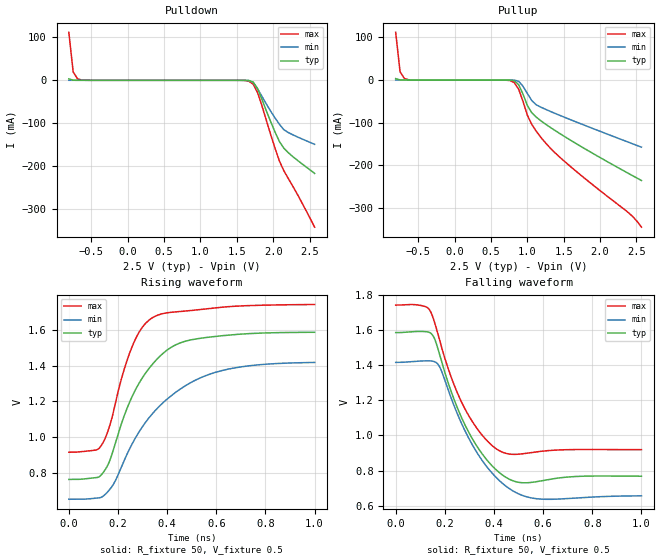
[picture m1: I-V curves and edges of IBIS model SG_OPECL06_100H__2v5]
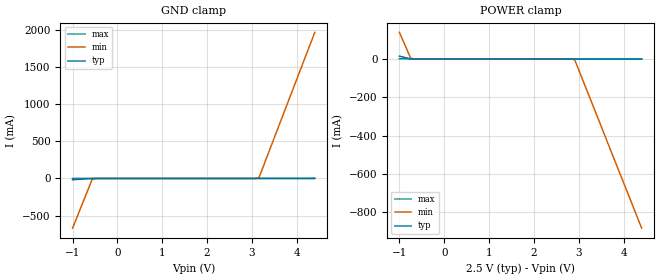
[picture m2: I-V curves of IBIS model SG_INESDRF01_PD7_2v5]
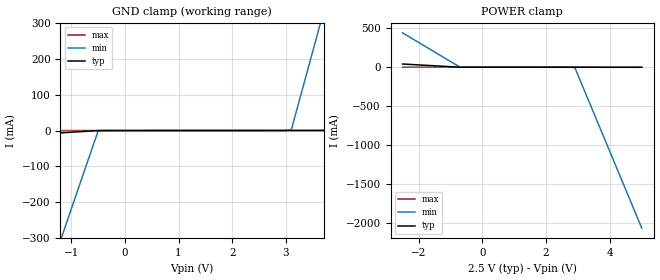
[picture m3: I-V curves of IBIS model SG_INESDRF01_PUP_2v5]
|   This file is an IBIS representation of the   |
|   Integrated Device Technology, INC   |
|   ICS853S013I   |
| LOW SKEW, DUAL, 1-TO-3, DIFFERENTIAL-TO-2.5V, 3.3V LVPECL/ECL FANOUT BUFFER  |
[IBIS Ver]   4.1
[File name]   853s013i.ibs
[File Rev]   1.0
[Date]   25 Aug 2010
[Source]   Originated at Integrated Device Technology, Inc.
[Disclaimer]
IDT hereby grants the user of this IBIS model a non-exclusive,
nontransferable license to use this IBIS model under the following terms.
Before using this IBIS model, the user should read this license.
If the user does not accept these terms,  the IBIS model should be
returned to IDT within 30 days.
   The user is granted this license only to use the IBIS model and
is not granted rights to sell, load, rent, lease or license the IBIS
model in whole or in part, or in modified form to anyone other than
user. User may modify the IBIS model to suit its specific
applications but rights to derivative works and such modifications
shall belong to IDT.
   This IBIS model is provided on an "AS IS" basis and IDT makes
absolutely no warranty with respect to the information contained
herein. IDT DISCLAIMS AND CUSTOMER WAIVES ALL WARRANTIES, EXPRESS
OR IMPLIED, INCLUDING WARRANTIES OF MERCHANTABILITY OR FITNESS FOR
A PARTICULAR PURPOSE. The entire risk as to quality and performance
is with the Customer. ACCORDINGLY, IN NO EVENT SHALL THE COMPANY BE
LIABLE FOR ANY DAMAGES, WHETHER IN CONTRACT OR TORT,INCLUDING ANY
LOST PROFITS OR OTHER INCIDENTAL, CONSEQUENTIAL, EXEMPLARY, OR
PUNITIVE DAMAGES ARISING OUT OF THE USE OR APPLICATION OF THE IBIS
model provided in this package. Further, IDT reserves the right to
make changes without notice to any product herein to improve
reliability, function, or design. IDT does not convey any license
under patent rights or any other intellectual property rights,
including those of third parties.
   IDT is not obligated to provide maintenance or support
for the licensed IBIS model.
[Copyright]   Copyright 2010 by Integrated Device Technology , Inc.
[Component]   ICS853S013MI
[Manufacturer] Integrated Device Technology, Inc.
[Package]
|SOIC 20 Lead
|   typ   min   max
R_pkg   57.15m   45.4m   68.9m
L_pkg   4.051n   2.187n   5.914n
C_pkg   0.796p   0.419p   1.173p
[Pin]   signal_name   model_name   R_pin   L_pin   C_pin
1   nQA0   SG_OPECL06_100H_   68.90m   5.914n   1.173p
2   QA0   SG_OPECL06_100H_   63.02m   4.983n   0.985p
3   VCC   POWER   57.15m   4.051n   0.796p
4   PCLKA   SG_INESDRF01_PD7   51.25m   3.119n   0.608p
5   nPCLKA  SG_INESDRF01_PUP   45.40m   2.187n   0.419p
6   PCLKB   SG_INESDRF01_PD7   45.40m   2.187n   0.419p
7   nPCLKB  SG_INESDRF01_PUP   51.25m   3.119n   0.608p
8   VCC   POWER   57.15m   4.051n   0.796p
9   nQB0   SG_OPECL06_100H_   63.02m   4.983n   0.985p
10   QB0   SG_OPECL06_100H_   68.90m   5.914n   1.173p
11   VEE   GND   68.90m   5.914n   1.173p
12   nQB1   SG_OPECL06_100H_   63.02m   4.983n   0.985p
13   QB1   SG_OPECL06_100H_   57.15m   4.051n   0.796p
14   nQB2   SG_OPECL06_100H_   51.25m   3.119n   0.608p
15   QB2   SG_OPECL06_100H_   45.40m   2.187n   0.419p
16   VCC   POWER   45.40m   2.187n   0.419p
17   nQA2   SG_OPECL06_100H_   51.25m   3.119n   0.608p
18   QA2   SG_OPECL06_100H_   57.15m   4.051n   0.796p
19   nQA1   SG_OPECL06_100H_   63.02m   4.983n   0.985p
20   QA1   SG_OPECL06_100H_   68.90m   5.914n   1.173p
[Diff Pin]  inv_pin  vdiff tdelay_typ tdelay_min  tdelay_max
2   1   NA   0   0   0
4   5   0.15   NA   NA   NA
6   7   0.15   NA   NA   NA
10   9   NA   0   0   0
13   12   NA   0   0   0
15   14   NA   0   0   0
18   17   NA   0   0   0
20   19   NA   0   0   0
[Model Selector] SG_OPECL06_100H_
SG_OPECL06_100H__2v5  Buffer selection for 2v5
SG_OPECL06_100H__3v3  Buffer selection for 3v3
[Model Selector] SG_INESDRF01_PD7
SG_INESDRF01_PD7_2v5  Buffer selection for 2v5
SG_INESDRF01_PD7_3v3  Buffer selection for 3v3
[Model Selector] SG_INESDRF01_PUP
SG_INESDRF01_PUP_2v5  Buffer selection for 2v5
SG_INESDRF01_PUP_3v3  Buffer selection for 3v3
| Models and submodels in the file (6): SG_OPECL06_100H__2v5 (Output_ECL), SG_INESDRF01_PD7_2v5 (Input), SG_INESDRF01_PUP_2v5 (Input), SG_OPECL06_100H__3v3 (Output_ECL), SG_INESDRF01_PD7_3v3 (Input), SG_INESDRF01_PUP_3v3 (Input)
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[Model] SG_OPECL06_100H__2v5
Model_type   Output_ECL
Polarity   Non-Inverting
|   typ   min   max
C_comp   2pF   1.5pF   2.5pF
Vmeas = 1.18V
Rref = 50
Cref = 0
Vref = 0.5V
|   typ   min   max
[Voltage range]   2.5V   2.375V   2.625V
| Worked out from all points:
|   rising waveform, R_fixture 50, V_fixture 0.5: 20-80 % time 168ps typ, 244ps min, 112ps max; typ from 0.766 V to 1.58 V
|   falling waveform, R_fixture 50, V_fixture 0.5: 20-80 % time 147ps typ, 166ps min, 138ps max; typ from 1.59 V to 0.768 V
[Pulldown]
|Voltage   I (typ)   I (min)   I (max)
|Note, modeling breaks down at 250mA and above.  This is well beyond the functional   |
|operating range of the device.  Should this scenario occur, catastrophic failure and   |
|possible damage to the device and/or board is of higher concern than the I-V curve   |
|behavior.  The IBIS checker will flag currents in excess of 10A with warnings.  Lines   |
|with currents in excess of 0.35 A have been commented out.  The points still remain|
|available to the user if the user desires to use them.   |
|-2.00000e+00   7.64199e+07   1.02823e+08   5.30176e+07
|-1.50000e+00   2.03995e+07   3.11849e+07   1.10674e+07
|-1.00000e+00   5.63549e+00   1.05412e+00   2.60079e+01
|-9.90000e-01   3.82790e+00   6.40804e-01   1.98508e+01
|-9.29670e-01   3.65720e-01   3.18126e-02   3.77220e+00
|-8.69341e-01   3.49411e-02   1.57933e-03   6.50010e-01
-809mV    3.338mA    78.41uA    112mA
-748.7mV  318.9uA    3.892uA    19.3mA
-688.4mV  30.47uA    193.3nA    3.326mA
-567.7mV  278.2nA    505.6pA    98.77uA
1.604V    -49.89uA   -23.57uA   -354.4uA
1.725V    -4.145mA   -5.161mA   -8.879mA
1.785V    -19.24mA   -19.54mA   -28.51mA
2.026V    -120.9mA   -88.02mA   -158.8mA
2.087V    -143.3mA   -102.8mA   -188.9mA
2.147V    -158.5mA   -115.4mA   -211mA
2.328V    -186mA     -131.8mA   -264.7mA
2.569V    -217.4mA   -149.5mA   -342.8mA
| 2.62978e+00   -2.26029e-01   -1.53936e-01   -3.65081e-01
| 2.69011e+00   -2.35268e-01   -1.58484e-01   -3.83382e-01
| 2.75044e+00   -2.44971e-01   -1.63081e-01   -3.98156e-01
| 2.81077e+00   -2.54678e-01   -1.67770e-01   -4.12183e-01
| 2.87110e+00   -2.64899e-01   -1.72632e-01   -4.26213e-01
| 2.93143e+00   -2.75604e-01   -1.77835e-01   -4.40413e-01
| 2.99176e+00   -2.86635e-01   -1.83484e-01   -4.54896e-01
| 3.05209e+00   -2.98827e-01   -1.89822e-01   -4.70365e-01
| 3.11242e+00   -3.12132e-01   -1.98614e-01   -4.93936e-01
| 3.17275e+00   -3.37194e-01   -2.38375e-01   -5.66611e-01
| 3.23308e+00   -4.99217e-01   -8.89863e-01   -9.25064e-01
| 3.29341e+00   -2.09975e+00   -1.15558e+01   -2.94227e+00
| 3.35374e+00   -1.50448e+01   -1.81946e+02   -1.21661e+01
| 3.41407e+00   -1.29054e+02   -3.55554e+03   -5.71608e+01
| 3.47440e+00   -1.29965e+03   -7.14273e+04   -3.09620e+02
| 3.53473e+00   -1.35272e+04   -9.09176e+05   -1.76605e+03
| 3.59505e+00   -1.41468e+05   -2.14513e+06   -1.02089e+04
| 3.65538e+00   -9.20284e+05   -4.24858e+06   -5.91895e+04
| 3.71571e+00   -1.86927e+06   -1.28417e+07   -3.43421e+05
| 3.77604e+00   -2.98794e+06   -2.26761e+07   -1.03824e+06
| 3.83637e+00   -5.88270e+06   -3.25106e+07   -1.74456e+06
| 3.89670e+00   -1.34687e+07   -4.23450e+07   -2.49457e+06
| 3.95703e+00   -2.11591e+07   -5.21795e+07   -3.49822e+06
| 4.01736e+00   -2.88496e+07   -6.20139e+07   -5.97377e+06
| 4.07769e+00   -3.65400e+07   -7.18484e+07   -1.16207e+07
| 4.13802e+00   -4.42304e+07   -8.16829e+07   -1.73796e+07
| 4.19835e+00   -5.19209e+07   -9.15173e+07   -2.31385e+07
| 4.25868e+00   -5.96113e+07   -1.01352e+08   -2.88974e+07
| 4.31901e+00   -6.73018e+07   -1.11186e+08   -3.46563e+07
| 4.37934e+00   -7.49922e+07   -1.21021e+08   -4.04152e+07
| 4.43967e+00   -8.26826e+07   -1.30855e+08   -4.61741e+07
| 4.50000e+00   -9.03731e+07   -1.40690e+08   -5.19330e+07
| 4.51000e+00   -9.16478e+07   -1.42320e+08   -5.28875e+07
| 4.67333e+00   -1.12468e+08   -1.68945e+08   -6.84789e+07
| 4.83667e+00   -1.33289e+08   -1.95570e+08   -8.40702e+07
| 5.00000e+00   -1.54110e+08   -2.22196e+08   -9.96615e+07
[Pullup]
|Voltage   I (typ)   I (min)   I (max)
|Note, modeling breaks down at 250mA and above.  This is well beyond the functional   |
|operating range of the device.  Should this scenario occur, catastrophic failure and   |
|possible damage to the device and/or board is of higher concern than the I-V curve   |
|behavior.  The IBIS checker will flag currents in excess of 10A with warnings.  Lines   |
|with currents in excess of 0.35 A have been commented out.  The points still remain|
|available to the user if the user desires to use them.   |
|-2.00000e+00   7.64199e+07   1.02823e+08   5.30176e+07
|-1.50000e+00   2.03995e+07   3.11849e+07   1.10674e+07
|-1.00000e+00   5.63549e+00   1.05412e+00   2.60079e+01
|-9.90000e-01   3.82790e+00   6.40804e-01   1.98508e+01
|-9.29670e-01   3.65720e-01   3.18126e-02   3.77220e+00
|-8.69341e-01   3.49411e-02   1.57933e-03   6.50010e-01
-809mV    3.338mA    78.41uA    112mA
-748.7mV  318.9uA    3.892uA    19.3mA
-688.4mV  30.47uA    193.3nA    3.326mA
699.2mV   -17.1uA    -493.3nA   -208.9uA
819.9mV   -1.608mA   -180.1uA   -5.692mA
880.2mV   -10.58mA   -2.702mA   -21.1mA
1.001V    -59.68mA   -31.46mA   -82.44mA
1.061V    -76.72mA   -48.04mA   -103.9mA
1.242V    -102.4mA   -68mA      -145.8mA
1.604V    -142.2mA   -93.71mA   -204.4mA
2.388V    -218.9mA   -145.7mA   -310.9mA
2.569V    -235.8mA   -157.5mA   -345.2mA
| 2.62978e+00   -2.41326e-01   -1.61350e-01   -3.60418e-01
| 2.69011e+00   -2.46895e-01   -1.65243e-01   -3.76659e-01
| 2.75044e+00   -2.52543e-01   -1.69143e-01   -3.93177e-01
| 2.81077e+00   -2.58498e-01   -1.73089e-01   -4.09370e-01
| 2.87110e+00   -2.65300e-01   -1.77128e-01   -4.25139e-01
| 2.93143e+00   -2.73435e-01   -1.81435e-01   -4.40333e-01
| 2.99176e+00   -2.82936e-01   -1.86258e-01   -4.54778e-01
| 3.05209e+00   -2.93556e-01   -1.91717e-01   -4.70091e-01
| 3.11242e+00   -3.06075e-01   -1.99317e-01   -4.93615e-01
| 3.17275e+00   -3.32122e-01   -2.37980e-01   -5.66272e-01
| 3.23308e+00   -4.95806e-01   -8.88645e-01   -9.24707e-01
| 3.29341e+00   -2.09737e+00   -1.15543e+01   -2.94188e+00
| 3.35374e+00   -1.50424e+01   -1.81945e+02   -1.21657e+01
| 3.41407e+00   -1.29051e+02   -3.55554e+03   -5.71603e+01
| 3.47440e+00   -1.29964e+03   -7.14273e+04   -3.09619e+02
| 3.53473e+00   -1.35272e+04   -9.09176e+05   -1.76605e+03
| 3.59505e+00   -1.41468e+05   -2.14513e+06   -1.02089e+04
| 3.65538e+00   -9.20284e+05   -4.24858e+06   -5.91895e+04
| 3.71571e+00   -1.86927e+06   -1.28417e+07   -3.43421e+05
| 3.77604e+00   -2.98794e+06   -2.26761e+07   -1.03824e+06
| 3.83637e+00   -5.88270e+06   -3.25106e+07   -1.74456e+06
| 3.89670e+00   -1.34687e+07   -4.23450e+07   -2.49457e+06
| 3.95703e+00   -2.11591e+07   -5.21795e+07   -3.49822e+06
| 4.01736e+00   -2.88496e+07   -6.20139e+07   -5.97377e+06
| 4.07769e+00   -3.65400e+07   -7.18484e+07   -1.16207e+07
| 4.13802e+00   -4.42304e+07   -8.16829e+07   -1.73796e+07
| 4.19835e+00   -5.19209e+07   -9.15173e+07   -2.31385e+07
| 4.25868e+00   -5.96113e+07   -1.01352e+08   -2.88974e+07
| 4.31901e+00   -6.73018e+07   -1.11186e+08   -3.46563e+07
| 4.37934e+00   -7.49922e+07   -1.21021e+08   -4.04152e+07
| 4.43967e+00   -8.26826e+07   -1.30855e+08   -4.61741e+07
| 4.50000e+00   -9.03731e+07   -1.40690e+08   -5.19330e+07
| 4.51000e+00   -9.16478e+07   -1.42320e+08   -5.28875e+07
| 4.67333e+00   -1.12468e+08   -1.68945e+08   -6.84789e+07
| 4.83667e+00   -1.33289e+08   -1.95570e+08   -8.40702e+07
| 5.00000e+00   -1.54110e+08   -2.22196e+08   -9.96615e+07
[Ramp]
|   typ   min   max
dV/dt_r   0.491/0.168n   0.456/0.243n   0.493/0.111n
dV/dt_f   0.517/0.161n   0.473/0.175n   0.512/0.146n
R_load =   50.0000
[Rising Waveform]
R_fixture = 50
V_fixture = 0.5   | VCC_typ - 2V
V_fixture_max = 0.625   | VCC_max - 2V
V_fixture_min = 0.375   | VCC_min - 2V
C_fixture = 0.0p
| Time   typ   min   max
0s        766.4mV    656.1mV    917.6mV
134.1ps   794.5mV    668.5mV    959.4mV
183.2ps   940.2mV    743.4mV    1.154V
218.2ps   1.093V     849.2mV    1.346V
255.3ps   1.221V     957.9mV    1.497V
295.3ps   1.323V     1.051V     1.605V
341.3ps   1.409V     1.134V     1.667V
441.4ps   1.519V     1.257V     1.699V
586.6ps   1.56V      1.358V     1.72V
1ns       1.585V     1.417V     1.739V
[Falling Waveform]
R_fixture = 50
V_fixture = 0.5   | VCC_typ - 2V
V_fixture_max = 0.625   | VCC_max - 2V
V_fixture_min = 0.375   | VCC_min - 2V
C_fixture = 0.0p
| Time   typ   min   max
0s        1.586V     1.416V     1.743V
117.1ps   1.592V     1.425V     1.736V
150.1ps   1.572V     1.423V     1.678V
182.2ps   1.443V     1.381V     1.526V
272.3ps   1.088V     1.055V     1.178V
343.3ps   911.7mV    875mV      1.016V
418.4ps   792.4mV    747.4mV    915.8mV
490.5ps   736mV      673.8mV    892.5mV
574.6ps   737.1mV    639.5mV    906.8mV
1ns       767.9mV    656.1mV    919.1mV
[Model] SG_INESDRF01_PD7_2v5
Model_type   Input
Polarity   Non-Inverting
Vinl = 0.7V
Vinh = 1.7V
|   typ   min   max
C_comp   2pF   1.5pF   2.5pF
|   typ   min   max
[Voltage range]   2.5V   2.375V   2.625V
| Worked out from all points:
|   GND clamp passes 1 mA (typ) near -0.58 V on its own axis
|   POWER clamp passes 1 mA (typ) near -0.76 V on its own axis
[GND_clamp]
|Voltage   I (typ)   I (min)   I (max)
-999mV    -17.25mA   -669.4mA   -57.61uA
-564.6mV  -245.6uA   -14.47mA   -7.295uA
-502.5mV  -27.9uA    -1.943mA   -6.234uA
3.035V    40.09uA    312uA      37.56uA
3.159V    51.32uA    15.14mA    39.1uA
4.4V      2.038mA    1.969A     54.5uA
[Power_clamp]
|Voltage   I (typ)   I (min)   I (max)
-999mV    14.5mA     139mA      411.1uA
-750.8mV  388.8uA    5.212mA    46.1uA
-688.7mV  72.95uA    733.8uA    41.21uA
2.787V    -3.782uA   -107uA     -1.999uA
2.911V    -6.009uA   -5.663mA   -3.535uA
4.4V      -171.1uA   -883.8mA   -21.97uA
[Model] SG_INESDRF01_PUP_2v5
Model_type   Input
Polarity   Non-Inverting
Vinl = 0.7V
Vinh = 1.7V
|   typ   min   max
C_comp   2pF   1.5pF   2.5pF
|   typ   min   max
[Voltage range]   2.5V   2.375V   2.625V
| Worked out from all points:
|   GND clamp passes 1 mA (typ) near -0.60 V on its own axis
|   POWER clamp passes 1 mA (typ) near -0.74 V on its own axis
[GND_clamp]
|Voltage   I (typ)   I (min)   I (max)
-2.5V     -18.68mA   -877.1mA   -176.4uA
-1.2V     -6.595mA   -308.2mA   -105.3uA
-1.1V     -5.665mA   -264.4mA   -99.8uA
-500mV    -88.13uA   -1.852mA   -66.99uA
3V        68.88uA    161.5uA    62.36uA
3.1V      73.77uA    2.321mA    66.06uA
3.6V      328.3uA    277.5mA    84.54uA
3.7V      379.2uA    332.6mA    88.23uA
5V        1.041mA    1.048A     136.3uA
[Power_clamp]
|Voltage   I (typ)   I (min)   I (max)
-2.5V     41.65mA    441.8mA    1.036mA
-700mV    124.7uA    1.074mA    74.72uA
2.9V      -65.32uA   -4.078mA   -58.67uA
5V        -544.4uA   -2.07A     -136.3uA
